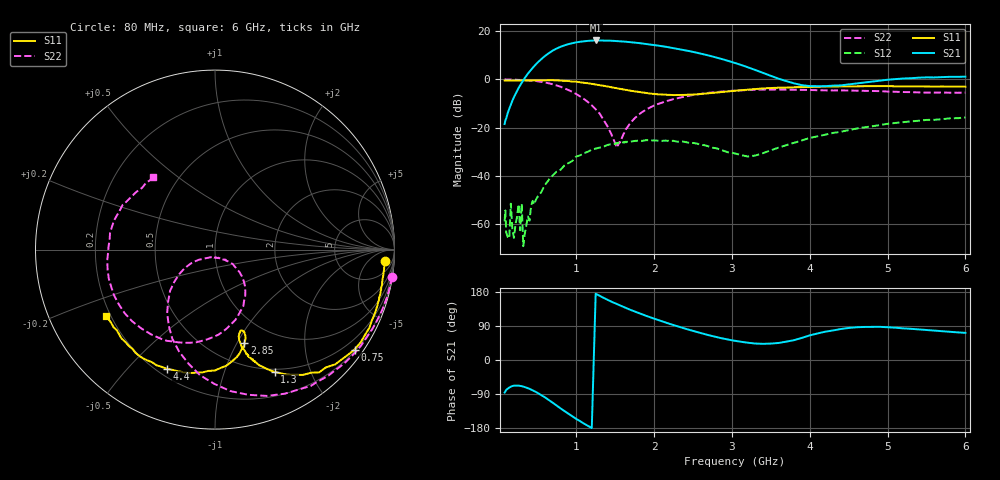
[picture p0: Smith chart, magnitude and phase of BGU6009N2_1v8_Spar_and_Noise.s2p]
! BGU6009N2, Vcc=1.8V, Icc= 5.2050 mA
# MHz S MA R 50
!  Freq-MHz  S11-mag  S11-arg  S21-mag  S21-arg  S12-mag  S12-arg  S22-mag  S22-arg
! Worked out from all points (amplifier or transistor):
!   130 points, 80 MHz to 6 GHz, reference 50 ohm
!   highest |S21| = 16.2 dB at 1.25 GHz (marker M1)
!   |S21| within 3 dB of that: 772.2 MHz to 2.218 GHz (1.446 GHz wide, 96.7 % of centre)
!   unconditionally stable (mu >= 1): 91.98 MHz to 158.7 MHz; 161.3 MHz to 998.6 MHz; 1.004 GHz to end of sweep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
!   at 480 MHz: K = 1.73, MAG = 23.1 dB, |S12| = -50.0 dB
!   at 1.615 GHz: K = 1.10, MAG = 18.8 dB, |S12| = -25.9 dB
!   at 6 GHz: K = 1.42, MAG = 4.6 dB, |S12| = -15.8 dB
!   lowest NFmin = 0.78 dB at 1 GHz
!   S11 on the Smith chart (normalised r, x): 80 MHz: 15, -18; 750 MHz: 0.24, -3.10; 1.3 GHz: 0.47, -1.50; 2.85 GHz: 0.72, -1.07; 4.4 GHz: 0.24, -0.65; 6 GHz: 0.18, -0.27
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80  0.9475 -3.7  0.119 -85.9  0.001141 -12.6  0.9978 -8.8
140  0.9477 -6.2  0.2471 -72.7  0.0005061 124.7  0.994 -15.5
160  0.9484 -6.9  0.2989 -70.4  0.002653 130.7  0.9917 -17.7
200  0.9485 -8.6  0.4291 -67.7  0.0005181 58.6  0.9875 -22.0
300  0.9496 -12.8  0.8543 -69.1  0.002654 -166.8  0.9736 -33.6
320  0.9523 -13.7  0.9624 -70.1  0.0003489 -24.1  0.9693 -35.9
480  0.9585 -20.7  2.035 -84.1  0.003148 171.8  0.9285 -55.0
750  0.9563 -35.6  4.381 -120.6  0.01229 173.9  0.7488 -90.2
900  0.9262 -43.7  5.399 -141.8  0.01836 161.4  0.602 -109.4
1100  0.8522 -55.0  6.168 -167.9  0.02958 136.7  0.3925 -131.8
1250  0.7857 -61.6  6.42 174.9  0.0368 126.5  0.2406 -145.7
1300  0.7587 -64.0  6.409 169.4  0.03864 121.6  0.1968 -148.6
1510  0.662 -70.3  6.263 148.7  0.04703 106.2  0.04262 -103.8
1700  0.5818 -73.8  5.912 132.0  0.05137 93.6  0.1277 -39.2
2100  0.4859 -73.9  4.891 102.1  0.0533 71.4  0.3286 -60.5
2450  0.4837 -70.8  3.874 79.7  0.04838 57.2  0.4577 -84.2
2850  0.5459 -72.5  2.707 58.2  0.03507 54.1  0.5554 -111.4
3100  0.5933 -76.5  2.04 48.6  0.02753 64.5  0.5915 -127.0
4100  0.7052 -104.0  0.7237 70.0  0.06616 110.1  0.5968 -177.9
4400  0.7166 -112.0  0.7529 81.8  0.08192 106.1  0.5921 171.1
5100  0.7195 -129.7  1.012 85.3  0.1253 93.8  0.554 148.8
6000  0.7084 -148.7  1.141 71.6  0.1628 77.9  0.5312 130.3
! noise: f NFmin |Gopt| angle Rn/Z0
1000  0.7818  0.3785  39.4  0.1801
1250  0.8507  0.3725  45.51  0.1714
1505  0.838  0.3631  50.8  0.1673
1535  0.8754  0.362  51.44  0.169
1560  0.8792  0.3626  52.23  0.1742
1590  0.8426  0.3505  54.2  0.169
1620  0.8479  0.3556  53.59  0.1674
1645  0.8449  0.3598  53.71  0.1671
1900  0.8712  0.365  59.68  0.1692
2200  0.9304  0.3693  66.76  0.1735
